FUNCTION_BLOCK FB_HRErrHist
(* v1.10
build up an error history consisting of two arrays and one index.
The index shows the actual array position. The last error id and the count for this id are saved in the arrays.
If an error id is the same as the previous input error the counter is increased. Otherwise the index is increased.
*)
VAR_INPUT
	bEdgeDetect	: BOOL;	(* FALSE: every input(bErr) is processed; TRUE: only rising edge of input is processed *)
END_VAR
VAR_OUTPUT
	nErrSum		: UINT;
	nErrIdx		: UINT; // error list index of last occured error (max. cHistLen)
	aErrList	: ARRAY[1..cHistLen] OF ST_HRErrHist;
END_VAR

VAR
	bNewErr		: BOOL;
	fbErrTrig	: R_TRIG;
END_VAR
VAR CONSTANT
	cHistLen	: UINT := 100;
END_VAR

METHOD AddError
VAR_INPUT
	bErr		: BOOL;
	hrErrCode	: HRESULT;
	sErrSource	: STRING(63);
END_VAR
fbErrTrig(CLK:=bErr);
IF bEdgeDetect THEN
	bNewErr := fbErrTrig.Q;
ELSE
	bNewErr := bErr;
END_IF

IF bNewErr THEN
	nErrSum := nErrSum + 1;
	IF nErrIdx < cHistLen THEN
		IF nErrIdx = 0 THEN
			nErrIdx	:= nErrIdx + 1;
		ELSIF aErrList[nErrIdx].hrErrCode <> hrErrCode OR aErrList[nErrIdx].sErrSource <> sErrSource THEN
			nErrIdx	:= nErrIdx + 1;
		END_IF
		aErrList[nErrIdx].hrErrCode := hrErrCode;
		aErrList[nErrIdx].sErrSource := sErrSource;
		aErrList[nErrIdx].nErrCount := aErrList[nErrIdx].nErrCount + 1;
	END_IF
END_IF
END_METHOD

METHOD Reset
VAR_INPUT
END_VAR
nErrSum := 0;
nErrIdx := 0;
MEMSET(ADR(aErrList),0,SIZEOF(aErrList));
END_METHOD

END_FUNCTION_BLOCK
